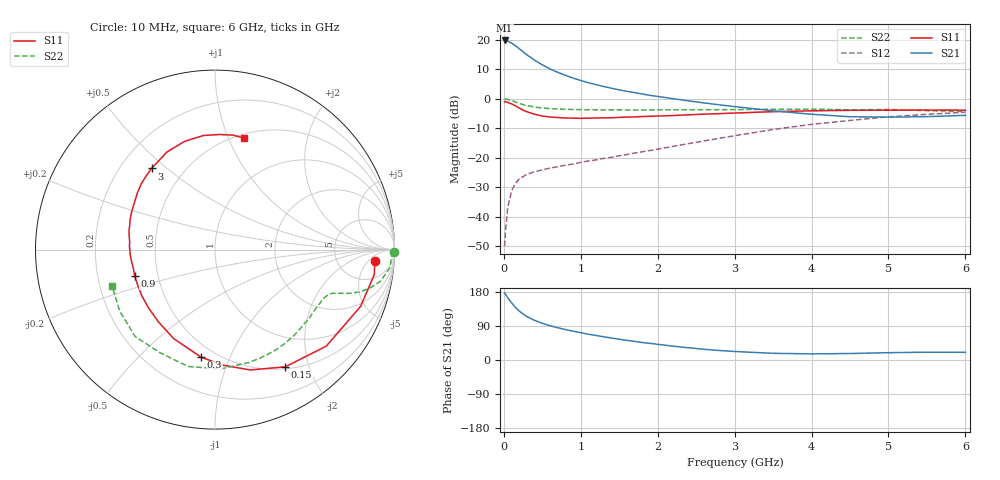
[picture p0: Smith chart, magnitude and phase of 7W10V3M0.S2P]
! Infineon Technologies  Discrete & RF Semiconductors
! BFS17W
! Si NPN RF Bipolar Junction Transistor in SOT323
! VCE = 10 V  IC = 3 mA
! Common Emitter S-Parameters:  August  1999
# GHz  S  MA  R  50
!  f  S11  S21  S12  S22
! GHz  MAG  ANG  MAG  ANG  MAG  ANG  MAG  ANG
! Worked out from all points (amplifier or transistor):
!   36 points, 10 MHz to 6 GHz, reference 50 ohm
!   highest |S21| = 19.8 dB at 10 MHz (marker M1)
!   |S21| within 3 dB of that: start of sweep to 210.1 MHz
!   unconditionally stable (mu >= 1): 742.5 MHz to 2.453 GHz; 5.09 GHz to end of sweep
!   at 250 MHz: K = 0.44, MSG = 21.1 dB, |S12| = -26.4 dB
!   at 1.4 GHz: K = 1.23, MAG = 8.8 dB, |S12| = -19.8 dB
!   at 6 GHz: K = 1.06, MAG = -2.0 dB, |S12| = -4.5 dB
!   S11 on the Smith chart (normalised r, x): 10 MHz: 12, -8; 150 MHz: 0.53, -1.64; 300 MHz: 0.42, -0.79; 900 MHz: 0.37, -0.14; 3 GHz: 0.33, +0.44; 6 GHz: 0.54, +1.14
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0.01  0.8924 -4.2  9.731 177.3  0.0032 79.3  0.9982 -0.7
0.02  0.8985 -8.9  9.726 173.7  0.0055 86.3  0.9843 -2.3
0.05  0.8707 -21.3  9.488 164.5  0.0144 77.1  0.9799 -5.9
0.1  0.8208 -40.9  8.776 151.0  0.0274 68.4  0.9386 -10.8
0.15  0.7614 -59.1  7.925 138.9  0.0368 61.0  0.8856 -14.2
0.2  0.6986 -73.7  7.064 129.3  0.044 56.4  0.8389 -16.3
0.25  0.6451 -86.2  6.238 121.4  0.0481 52.0  0.7981 -17.7
0.3  0.6045 -97.3  5.561 114.9  0.0528 49.8  0.7689 -18.5
0.4  0.5467 -114.9  4.511 104.6  0.0582 47.5  0.7245 -19.6
0.5  0.5109 -128.2  3.762 96.9  0.0628 46.9  0.7002 -20.3
0.6  0.4922 -139.2  3.211 90.5  0.0672 47.9  0.6831 -21.3
0.7  0.4822 -147.8  2.811 85.2  0.0709 49.5  0.6725 -22.6
0.9  0.471 -162.0  2.243 76.1  0.0789 52.6  0.6592 -25.4
1.1  0.4702 -172.9  1.874 68.0  0.0887 55.8  0.6525 -28.9
1.3  0.4767 177.9  1.615 61.2  0.0982 59.2  0.6485 -32.8
1.6  0.4915 167.0  1.336 51.8  0.1141 63.1  0.6467 -39.0
2.2  0.5212 149.1  1.004 36.5  0.1568 69.7  0.6518 -53.0
3  0.5741 128.0  0.738 22.5  0.2372 71.6  0.6568 -73.2
3.5  0.6061 116.2  0.626 17.6  0.3019 69.1  0.6656 -87.3
4.5  0.6389 95.8  0.497 17.1  0.4304 57.7  0.6512 -118.0
5.5  0.6458 81.1  0.499 20.6  0.5468 44.1  0.6316 -147.3
6  0.6416 75.5  0.525 20.4  0.5926 37.3  0.6079 -160.5
